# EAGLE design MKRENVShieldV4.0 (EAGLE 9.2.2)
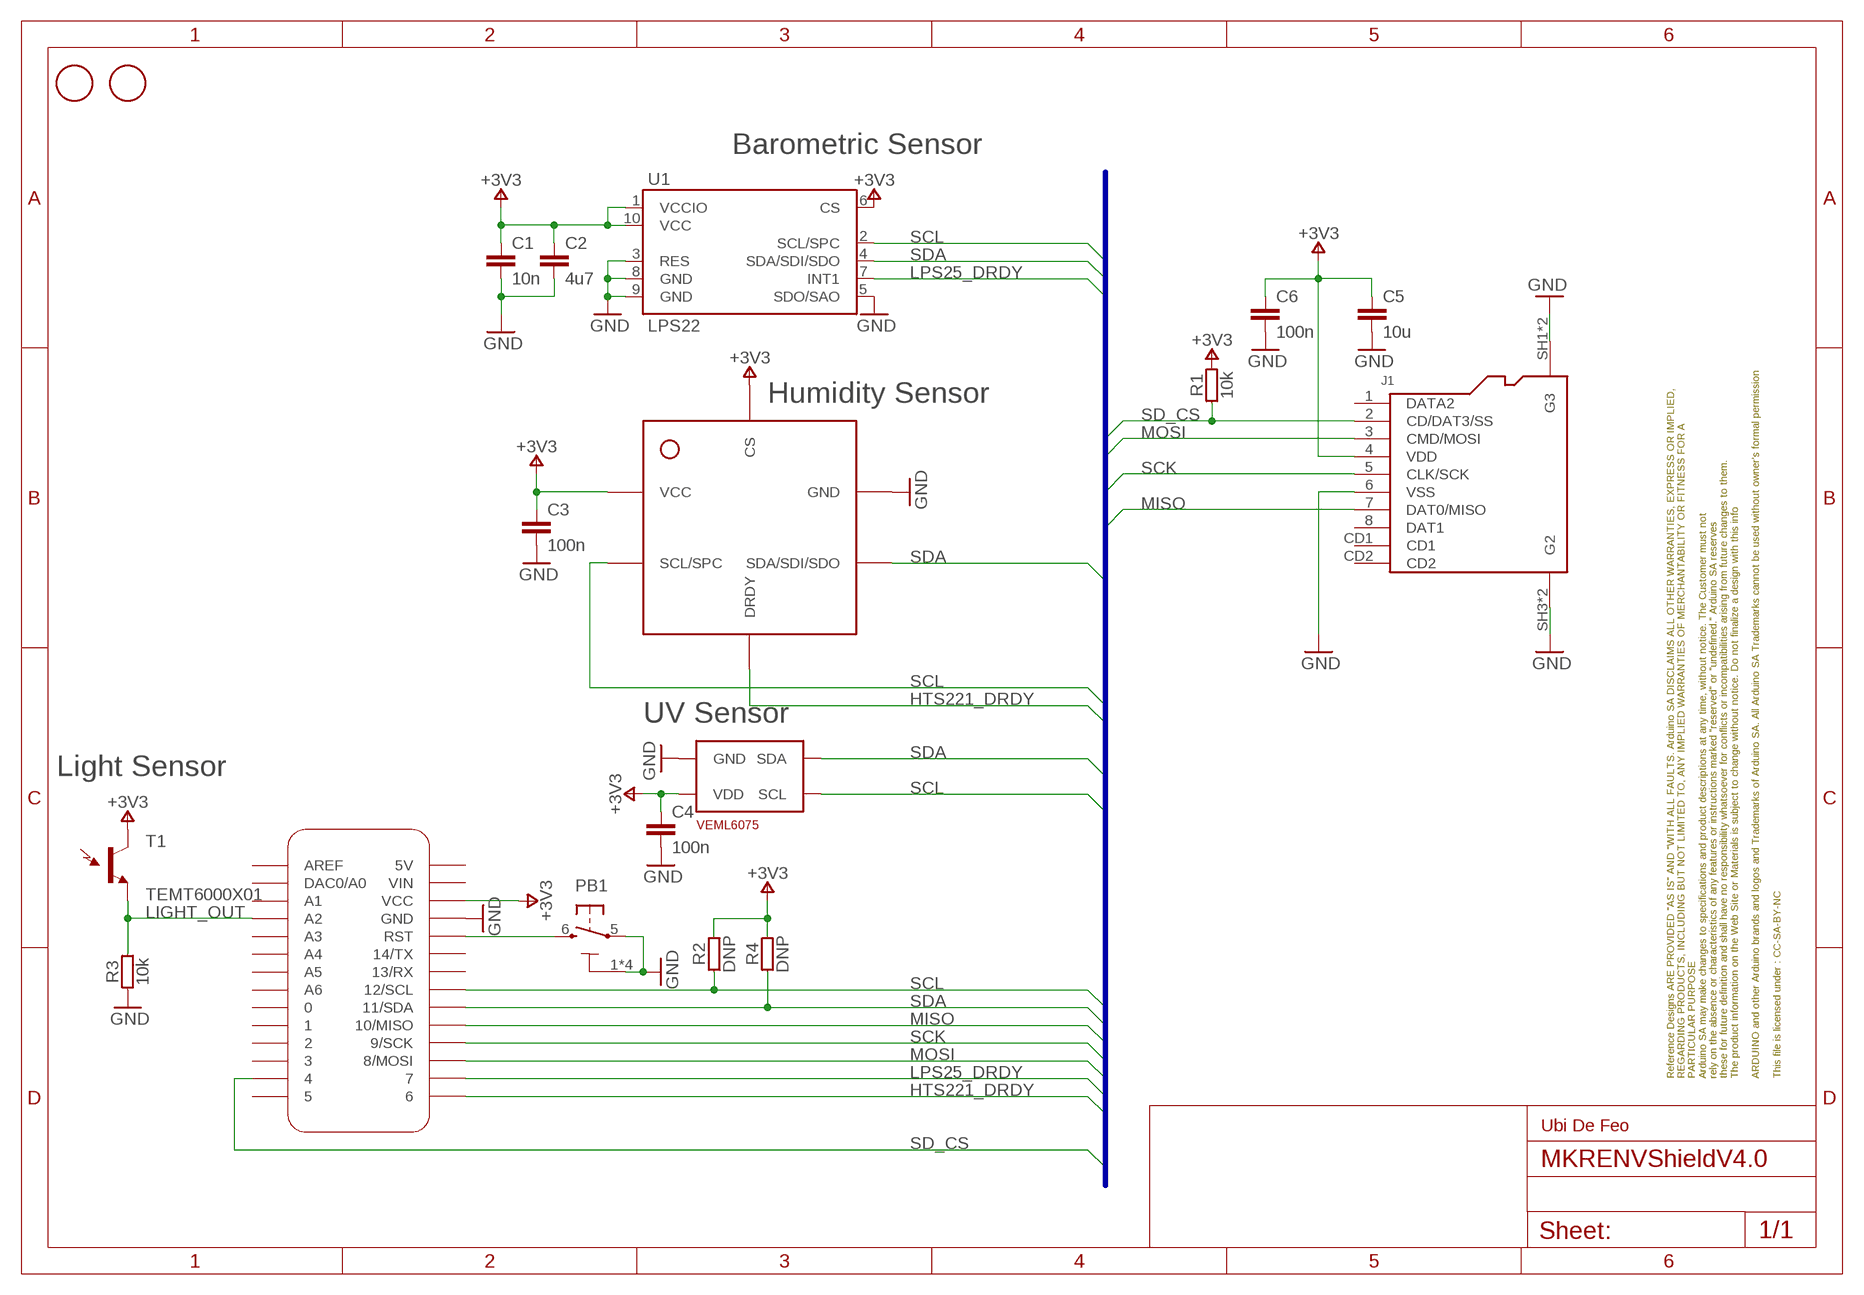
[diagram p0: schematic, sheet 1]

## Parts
C1  10n  C-10NF-0402  [0402-1005X55N]
C2  4u7  C-4.7UF-0402  [0402-1005X55N]
C3  100n  C-100NF-0402  [0402-1005X55N]
C4  100n  C-100NF-0402  [0402-1005X55N]
C5  10u  C-10UF-0603  [0603-1608X90N]
C6  100n  C-100NF-0402  [0402-1005X55N]
FD1  DNP  FIDUCIAL-1.5MM  [FD-1-1.5]
FD2  DNP  FIDUCIAL-1.5MM  [FD-1-1.5]
FRAME1  DNP  A4L-LOC  [FRAME]
J1  -  SD_AMPHENOL  [AMPHENOL_114-00841-68]
MKR1  -  MKRBOARD-SHORTTEXT  [MKRBOARD-DIM-SHORTTEXT]
PB1  PTS820  TACTILE1PTS820-NH  [C&K_PTS820_NO_HOLES]
R1  10k  R-10K-0402  [0402-1005X55N]
R2  DNP  R-DNP-0402  [0402-1005X55N]
R3  10k  R-10K-0402  [0402-1005X55N]
R4  DNP  R-DNP-0402  [0402-1005X55N]
T1  TEMT6000X01  TEMT6000  [TEMT6000-SEN]
U1  LPS22  LPS2XH-22  [LPS22H]
U2  HTS221  [HTS221]
U4  VEML6075  [VEML6075]

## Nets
+3V3: C1.1 C2.1 C3.1 C4.1 C5.1 C6.1 J1.4(VDD) MKR1.VCC R1.2 R2.2 R4.2 T1.COLLECTOR(C1) U1.1(VCCIO) U1.6(CS) U1.10(VCC) U2.P$1.VDD(VCC) U2.P$6.CS(CS) U4.P$4(VDD)
GND: C1.2 C2.2 C3.2 C4.2 C5.2 C6.2 J1.6(VSS) J1.SH1(G3) J1.SH2(G3) J1.SH3(G2) J1.SH4(G2) MKR1.GND PB1.1 PB1.2 PB1.3 PB1.4 PB1.5 R3.1 U1.3(RES) U1.5(SDO/SAO) U1.8(GND) U1.9(GND) U2.P$5.GND(GND) U4.P$1(GND)
HTS221_DRDY: MKR1.6 U2.P$3.DRDY(DRDY)
LIGHT_OUT: MKR1.A2 R3.2 T1.EMITTER(E1)
LPS25_DRDY: MKR1.7 U1.7(INT1)
MISO: J1.7(DAT0/MISO) MKR1.10(10/MISO)
MOSI: J1.3(CMD/MOSI) MKR1.8(8/MOSI)
RESET: MKR1.RST PB1.6
SCK: J1.5(CLK/SCK) MKR1.9(9/SCK)
SCL: MKR1.12(12/SCL) R2.1 U1.2(SCL/SPC) U2.P$2.SCL/SPC(SCL/SPC) U4.P$3(SCL)
SD_CS: J1.2(CD/DAT3/SS) MKR1.4 R1.1
SDA: MKR1.11(11/SDA) R4.1 U1.4(SDA/SDI/SDO) U2.P$4.SDA/SDI/SDO(SDA/SDI/SDO) U4.P$2(SDA)
Unconnected: J1.1(DATA2) J1.8(DAT1) J1.CD1 J1.CD2 MKR1.0 MKR1.1 MKR1.2 MKR1.3 MKR1.5 MKR1.5V MKR1.13(13/RX) MKR1.14(14/TX) MKR1.A0(DAC0/A0) MKR1.A1 MKR1.A3 MKR1.A4 MKR1.A5 MKR1.A6 MKR1.AREF MKR1.VIN

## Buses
HTS221_DRDY,LPS25_DRDY,MISO,MOSI,SCK,SCL,SDA,SD_CS

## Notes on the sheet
- Barometric Sensor
- Humidity Sensor
- UV Sensor
- Light Sensor
- Ubi De Feo

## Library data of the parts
C1 = Arduino-rcl:C: SMD Capacitor; CODE-ARDUINO: 0165; DATASHEET: http://search.murata.co.jp/Ceramy/image/img/A01X/partnumbering_e_01.pdf; DISTRIBUTOR-LINK: http://www.digikey.com/product-detail/en/murata-electronics-north-america/GRM155R71H103KA88J/490-6351-1-ND/3845548; DISTRIBUTOR-PN: 490-6351-1-ND; MANUFACTURER: Murata; MANUFACTURER-PN: GRM155R71H103KA88J; NOTE: -
C2 = Arduino-rcl:C: SMD Capacitor; CODE-ARDUINO: 0833; DATASHEET: http://search.murata.co.jp/Ceramy/image/img/A01X/partnumbering_e_01.pdf; DISTRIBUTOR-LINK: http://www.digikey.com/product-detail/en/murata-electronics-north-america/GRM155R60J475ME47D/490-5915-1-ND/3719860; DISTRIBUTOR-PN: 490-5915-1-ND; MANUFACTURER: Murata; MANUFACTURER-PN: GRM155R60J475ME47D; NOTE: -
C3 C4 C6 = Arduino-rcl:C: SMD Capacitor; CODE-ARDUINO: 0132; DATASHEET: http://www.tdk.com/pdf/TDKMLCCCapRange.pdf; DISTRIBUTOR-LINK: http://www.digikey.com/product-detail/en/tdk-corporation/C1005X5R1H104K050BB/445-5942-1-ND/2443982; DISTRIBUTOR-PN: 445-5942-1-ND; MANUFACTURER: TDK; MANUFACTURER-PN: C1005X5R1H104K050BB; NOTE: -
C5 = Arduino-rcl:C: SMD Capacitor; CODE-ARDUINO: 2213; DATASHEET: http://www.murata.com/~/media/webrenewal/support/library/catalog/products/capacitor/mlcc/c02e.pdf; DISTRIBUTOR-LINK: http://www.digikey.com/product-search/en?keywords=490-10728-1-ND; DISTRIBUTOR-PN: 490-10728-1-ND; MANUFACTURER: Murata; MANUFACTURER-PN: GRM188R61C106KAALD; NOTE: -
FD1 FD2 = Arduino-utility:FIDUCIAL: Fiducial mount; CODE-ARDUINO: DNP; DATASHEET: DNP; DISTRIBUTOR-LINK: DNP; DISTRIBUTOR-PN: DNP; MANUFACTURER: DNP; MANUFACTURER-PN: DNP
FRAME1 = Arduino-utility:A4L-LOC: FRAME; CODE-ARDUINO: DNP; DATASHEET: DNP; DISTRIBUTOR-LINK: DNP; DISTRIBUTOR-PN: DNP; MANUFACTURER: DNP; MANUFACTURER-PN: DNP
J1 = Arduino-connectors:SD_AMPHENOL: Micro SD connector; CODE-ARDUINO: A5328; DATASHEET: https://www.amphenolcanada.com/ProductSearch/drawings/AC/1140084168.pdf; DISTRIBUTOR-LINK: http://www.digikey.com/product-detail/en/amphenol-commercial-products/114-00841-68/114-00841-68-1-ND/2187101; DISTRIBUTOR-PN: 114-00841-68-1-ND; MANUFACTURER: Amphenol; MANUFACTURER-PN: 114-00841-68; NOTE: NO
MKR1 = Arduino-utility:MKRBOARD: MKR board footprint; CODE-ARDUINO: -; DATASHEET: -; DISTRIBUTOR-LINK: -; DISTRIBUTOR-PN: -; MANUFACTURER: -; MANUFACTURER-PN: -
PB1 = Arduino-pushbuttons:TACTILE1: Tactile Switch SPST-NO Top Actuated Surface Mount; CODE-ARDUINO: 0173; DATASHEET: http://www.ckswitches.com/media/1474/pts820.pdf; DISTRIBUTOR-LINK: https://www.digikey.com/product-detail/en/c-k/PTS820-J15M-SMTR-LFS/CKN10506CT-ND/4176681; DISTRIBUTOR-PN: PTS820 J25K SMTR LFS-ND; MANUFACTURER: C&K; MANUFACTURER-PN: PTS820 J25K SMTR LFS
R1 R3 = Arduino-rcl:R: SMD Resistor; CODE-ARDUINO: 0136; DATASHEET: www.yageo.com.tw/exep/pages/download/literatures/PYu-R_INT-thick_7.pdf; DISTRIBUTOR-LINK: http://www.digikey.com/product-detail/en/yageo/RC0402FR-0710KL/311-10.0KLRCT-ND/729470; DISTRIBUTOR-PN: 311-10.0KLRCT-ND; MANUFACTURER: Yageo; MANUFACTURER-PN: RC0402FR-0710KL; NOTE: NO
R2 R4 = Arduino-rcl:R: SMD Resistor; CODE-ARDUINO: DNP; DATASHEET: DNP; DISTRIBUTOR-LINK: DNP; DISTRIBUTOR-PN: DNP; MANUFACTURER: DNP; MANUFACTURER-PN: DNP; NOTE: NO
T1 = Arduino-Sensors:TEMT6000: Ambient Light Sensor; CODE-ARDUINO: A5355; DATASHEET: https://www.vishay.com/docs/81579/temt6000.pdf; DISTRIBUTOR-LINK: https://nl.mouser.com/ProductDetail/Vishay-Semiconductors/TEMT6000X01?qs=sGAEpiMZZMtIHXa%252bTo%2fr2WJrbra4XIks; DISTRIBUTOR-PN: 78-TEMT6000; MANUFACTURER: Vishay Semiconductors; MANUFACTURER-PN: TEMT6000X01
U1 = Arduino-Sensors:LPS2XH; CODE-ARDUINO: A5390; DATASHEET: https://www.st.com/content/ccc/resource/technical/document/datasheet/bf/c1/4f/23/61/17/44/8a/DM00140895.pdf/files/DM00140895.pdf/jcr:content/translations/en.DM00140895.pdf; DISTRIBUTOR-LINK: https://www.digikey.com/product-detail/en/stmicroelectronics/LPS22HBTR/497-16265-1-ND/5799917; DISTRIBUTOR-PN: 497-16265-1-ND; MANUFACTURER: ST; MANUFACTURER-PN: LPS22HBTR
U2 = Arduino-Sensors:HTS221; CODE-ARDUINO: A5356; DATASHEET: https://nl.mouser.com/datasheet/2/389/hts221-954783.pdf; DISTRIBUTOR-LINK: https://nl.mouser.com/ProductDetail/STMicroelectronics/HTS221TR?qs=%2fha2pyFaduhYqhgVSCoMJjbIcKdCD1D5p03chi4OA3k%3d; DISTRIBUTOR-PN: 511-HTS221TR; MANUFACTURER: STMicroelectronics; MANUFACTURER-PN: HTS221TR
U4 = Arduino-Sensors:VEML6075: The VEML6075 senses UVA and UVB light and incorporates photodiode, amplifiers, and analog / digital circuits into a single chip using a CMOS process. When the UV sensor is applied, it is able to detect UVA and UVB intensity to provide a measure of the signal strength as well as allowing for UVI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; CODE-ARDUINO: A5354; DATASHEET: http://www.vishay.com/docs/84304/veml6075.pdf; DISTRIBUTOR-LINK: https://www.digikey.com/product-detail/en/vishay-semiconductor-opto-division/VEML6075/VEML6075CT-ND/5878946; DISTRIBUTOR-PN: VEML6075CT-ND; MANUFACTURER: Vishay Semiconductor Opto Division; MANUFACTURER-PN: VEML6075

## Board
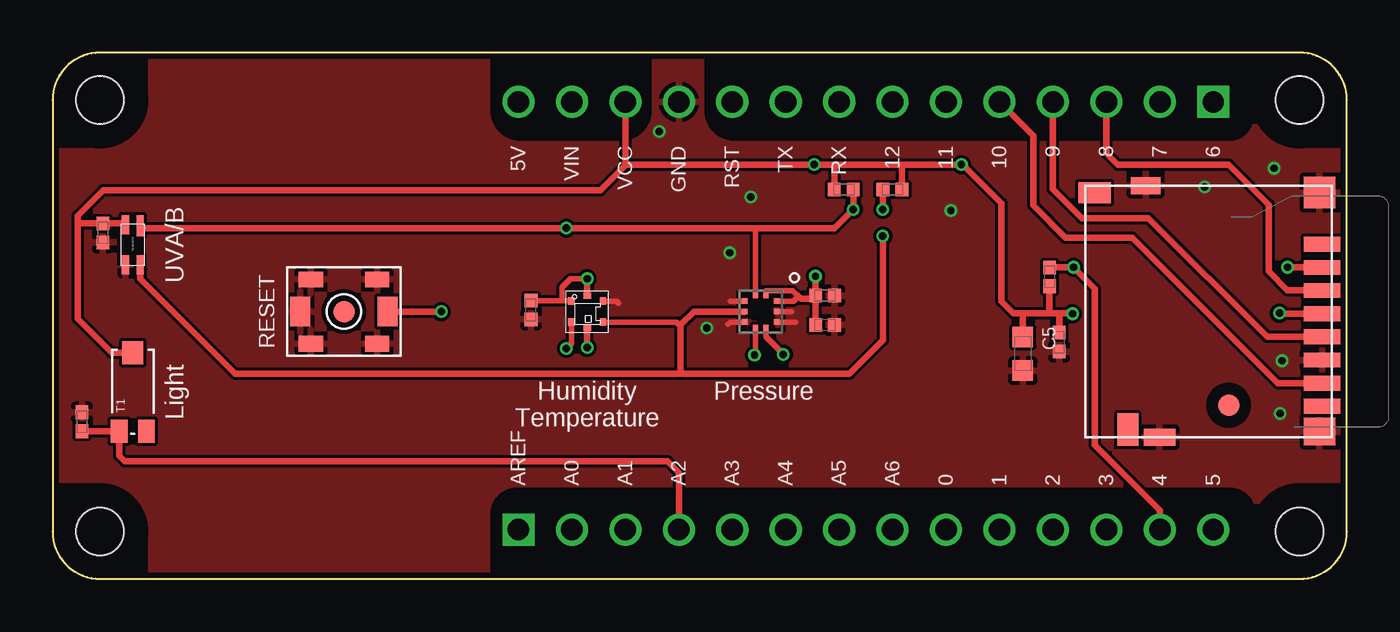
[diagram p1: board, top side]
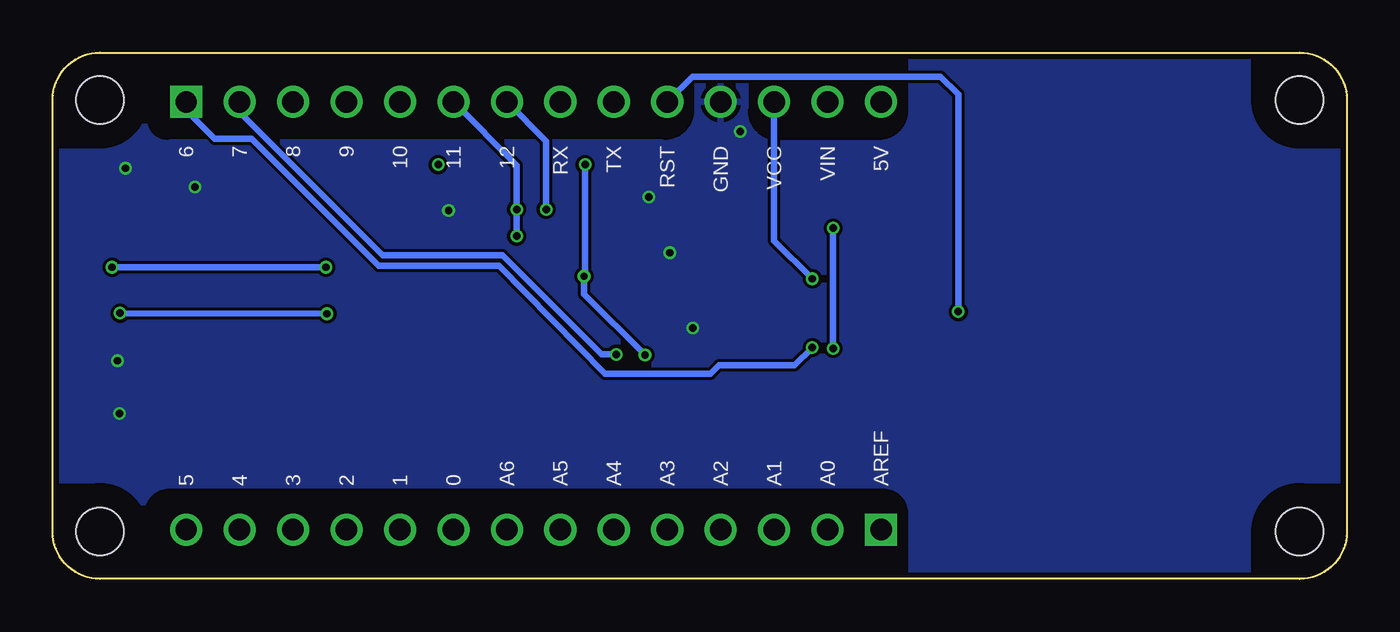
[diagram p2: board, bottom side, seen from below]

Size 61.5 x 25 mm. Coordinates in mm from the lower left corner, seen from the top.
Copper layers (1*16): Top 0.018mm / dielectric 1.55mm / Bottom 0.018mm
Design rules "eC_2Layer_PClass6_BaseCopperO18_eCDefault": minimum track width 0.15mm, minimum drill 0.35mm, track to track 0.15mm, track to pad 0.15mm, pad to pad 0.15mm, via to via 0.15mm, smd to smd 0mil, copper to edge 0.25mm, drill to drill 0.35mm, minimum pad ring 0.175mm, minimum via ring 0.125mm, stop-mask expansion 0mil, vias tented up to drill 0.45mm, thermal gap 0.2mm
tRestrict: area 33.2,12.3 to 34.1,13.1; area 32.5,13 to 33.1,13.7; area 32.5,11.7 to 33,12.3; area 24.4,11.7 to 26.4,13.7; area 3.1,14.9 to 4.4,16.9; 19 lines
bRestrict: 16 lines

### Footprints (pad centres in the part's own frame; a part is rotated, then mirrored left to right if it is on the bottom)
0402-1005X55N = smd 0.62 x 0.62: 1 -0.45,0; 2 0.45,0
0603-1608X90N = smd 0.95 x 1: 1 -0.8,0; 2 0.8,0
FD-1-1.5 = smd 1.016 x 1.016: P$1 0,0
AMPHENOL_114-00841-68 = smd 0.7 x 1.75: 1 3.2,-5.888; 2 2.1,-5.888; 3 1,-5.888; 4 -0.1,-5.888; 5 -1.2,-5.888; 6 -2.3,-5.888; 7 -3.4,-5.888; 8 -4.5,-5.888 | smd 1 x 1.55: CD1 5.65,4.912 | smd 1.55 x 1: CD2 -5.602,3.337 | smd 1.3 x 1.5: SH1 -5.7,-5.76 | smd 1.5 x 1.5: SH2 5.65,-5.76 | smd 0.8 x 1.4: SH3 5.975,2.487 | smd 0.8 x 1.5: SH4 -5.975,1.837
MKRBOARD-DIM-SHORTTEXT = drill 1.016 pad 1.524: 0 42.455,2.34; 1 44.995,2.34; 2 47.535,2.34; 3 50.075,2.34; 4 52.615,2.34; 5 55.155,2.34; 5V 22.135,22.66; 7 52.615,22.66; 8 50.075,22.66; 9 47.535,22.66; 10 44.995,22.66; 11 42.455,22.66; 12 39.915,22.66; 13 37.375,22.66; 14 34.835,22.66; A0 24.675,2.34; A1 27.215,2.34; A2 29.755,2.34; A3 32.295,2.34; A4 34.835,2.34; A5 37.375,2.34; A6 39.915,2.34; GND 29.755,22.66; RST 32.295,22.66; VCC 27.215,22.66; VIN 24.675,22.66 | drill 1.016 pad 1.524 square: 6 55.155,22.66; AREF 22.135,2.34 | hole 2.25: 59.25,2.25; 59.25,22.75; 2.25,2.25; 2.25,22.75
C&K_PTS820_NO_HOLES = smd 1.15 x 0.75: 1 -1.575,1.525; 2 -1.575,-1.525; 3 1.575,1.525; 4 1.575,-1.525 | smd 0.95 x 1.4: 5 -2.075,0; 6 2.075,0
TEMT6000-SEN = smd 1.1 x 0.8: BASE -1.87,-0.65; EMITTER -1.87,0.65 | smd 1.1 x 1: COLLECTOR 1.86,0.01
LPS22H = smd 0.25 x 0.275: 1 -0.25,-0.762; 2 0.25,-0.762; 6 0.25,0.762; 7 -0.25,0.762 | smd 0.275 x 0.25: 3 0.762,-0.5; 4 0.762,0; 5 0.762,0.5; 8 -0.762,0.5; 9 -0.762,0; 10 -0.762,-0.5
HTS221 = smd 0.3 x 0.35: P$1.VDD -0.75,0.5; P$2.SCL/SPC -0.75,-0.5; P$4.SDA/SDI/SDO 0.75,-0.5; P$5.GND 0.75,0.5 | smd 0.35 x 0.3: P$3.DRDY 0,-0.75; P$6.CS 0,0.75
VEML6075 = smd 0.9 x 0.35: P$1 -0.95,0.35; P$2 -0.95,-0.35; P$4 0.95,0.35 | smd 1 x 0.35: P$3 0.9,-0.35

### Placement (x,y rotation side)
C1  36.7,12.06 0 top
C2  36.7,13.46 0 top
C3  22.73,12.78 270 top
C4  2.39,16.43 270 top
C5  46.1,10.69 270 top
C6  47.83,11.25 270 top
FD1  13.84,12.7 0 top
FD2  55.88,8.26 0 top
FRAME1  not placed on the board
J1  54.43,12.7 90 top
MKR1  0,0 0 top
PB1  13.84,12.7 0 top
R1  47.37,14.35 270 top
R2  37.59,18.49 180 top
R3  1.4,7.47 270 top
R4  39.9,18.49 0 top
T1  3.81,8.89 90 top
U1  33.65,12.7 180 top
U2  25.4,12.7 0 top
U4  3.81,15.88 90 top

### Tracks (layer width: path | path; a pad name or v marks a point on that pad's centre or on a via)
+3V3  (via drill 0.35, 0.35 pad 0.25)
  Top 0.254: U1.6 33.4,10.68 v33.35,10.64 | U1.10 35.21,13.2 35.43,13.43 35.16,13.7 33.9,13.7 U1.1 | 24.2,13.23 C3.1 22.73,13.39 | 24.2,13.23 24.62,13.23 U2.P$1.VDD | v25.4,14.26 24.6,14.26 24.2,13.86 24.2,13.23
  Top 0.305: C2.1 36.09,13.3 35.56,13.3 35.43,13.43 | C1.1 C2.1 | C2.1 v36.25,14.38 | 37.08,19.68 v36.2,19.68 27.25,19.68 | 37.08,19.68 40.39,19.68 | 40.39,19.68 v43.18,19.68 43.25,19.68 45.09,17.85 45.09,13.18 45.64,12.62 46.1,12.62 | 47.83,12.62 47.45,12.62 | MKR1.VCC 27.21,19.72 27.25,19.68 | T1.COLLECTOR 2.81,10.75 1.19,12.37 1.19,16.87 | U2.P$6.CS v25.4,14.26 | J1.4 58.32,12.6 v58.29,12.62 | R2.2 37.14,19.63 37.08,19.68 | R4.2 40.35,19.65 40.39,19.68 | 27.25,19.68 26.04,18.47 2.42,18.47 1.19,17.25 1.19,16.87 | 1.19,16.87 1.21,16.88 C4.1 3.4,16.88 U4.P$4 | C6.1 47.83,12.62 | R1.2 47.37,12.7 47.45,12.62 | 47.45,12.62 46.1,12.62 | C5.1 46.1,12.62 | 47.83,12.62 48.44,12.62 v48.46,12.6
  Bottom 0.305: v48.46,12.6 v58.29,12.62 | v33.35,10.64 36.25,13.53 v36.25,14.38 36.2,14.43 v36.2,19.68 | v25.4,14.26 27.21,16.07 MKR1.VCC
GND  (via drill 0.35)
  Top 0.254: U1.8 35.3,12.2 | U1.9 35.1,12.7 | U1.3 32.2,13.2 | U1.5 32.2,12.2 32.1,12.1 | U2.P$5.GND 26.8,13.2 26.9,13.1
  other vias: 31.09,11.91 28.83,21.26 54.74,18.62 32.18,15.49 58.04,19.51 58.42,10.36 33.17,18.14 42.68,17.49 58.32,7.86
  pour Top: 2.54,25.02 59.18,25.02 arc-90 61.72,22.48 61.72,2.54 arc-90 59.18,0 2.54,0 arc-90 0,2.54 0,22.48 arc-90
  pour Bottom: 2.54,25.02 59.18,25.02 arc-90 61.72,22.48 61.72,2.54 arc-90 59.18,0 2.54,0 arc-90 0,2.54 0,22.48 arc-90
HTS221_DRDY  (via drill 0.35)
  Top 0.305: U2.P$3.DRDY v25.4,10.99
  Bottom 0.305: MKR1.6 55.16,22.27 53.81,20.92 52.03,20.92 46,14.89 40.29,14.89 35.26,9.73 30.23,9.73 29.83,10.14 26.25,10.14 v25.4,10.99
LIGHT_OUT
  Top 0.305: R3.2 T1.EMITTER 3.16,5.86 3.43,5.59 29.21,5.59 29.75,5.04 MKR1.A2
LPS25_DRDY  (via drill 0.35)
  Top 0.254: U1.7 33.9,11.49 v34.72,10.67
  Bottom 0.305: v34.72,10.67 35.42,10.67 40.13,15.38 45.83,15.38 52.62,22.16 MKR1.7
MISO
  Top 0.305: MKR1.10 46.6,21.06 46.6,17.75 48.13,16.21 51.31,16.21 58.22,9.3 J1.7
MOSI
  Top 0.305: MKR1.8 50.08,20.23 50.62,19.68 55.88,19.68 57.78,17.78 57.78,14.61 58.67,13.72 60.3,13.72 J1.3
RESET  (via drill 0.35)
  Top 0.305: PB1.6 v18.47,12.7
  Bottom 0.305: v18.47,12.7 18.47,23.01 19.3,23.85 31.1,23.85 MKR1.RST
SCK
  Top 0.305: MKR1.9 47.53,18.5 48.9,17.14 52.07,17.14 57.72,11.5 J1.5
SCL  (via drill 0.35)
  Top 0.254: U1.2 33.4,16.62 33.35,16.66 | U2.P$2.SCL/SPC 24.65,11.19 v24.41,10.95
  Top 0.305: R2.1 v38.04,17.56 | v38.04,17.56 v38.05,17.55 | 33.35,16.66 v24.41,16.66 4.27,16.66 U4.P$3 | 33.35,16.66 37.15,16.66 v38.04,17.56 | 33.35,16.66
  Bottom 0.305: MKR1.12 38.05,20.79 v38.05,17.55 | v24.41,16.66 v24.41,10.95
SD_CS  (via drill 0.35)
  Top 0.305: R1.1 v48.51,14.81 49.53,13.79 49.53,6.35 52.62,3.27 MKR1.4 | J1.2 58.68,14.8 v58.67,14.81
  Bottom 0.305: v58.67,14.81 v48.51,14.81
SDA  (via drill 0.35)
  Top 0.254: 29.84,12 29.64,12.2 U2.P$4.SDA/SDI/SDO
  Top 0.305: U1.4 30.48,12.7 29.84,12.06 29.84,12 29.84,9.79 29.8,9.74 | v39.45,16.28 39.47,16.26 39.47,11.34 37.87,9.73 29.83,9.73 29.83,9.74 29.8,9.74 | R4.1 v39.45,17.55 | U4.P$2 4.16,14.26 8.67,9.74 29.8,9.74
  Bottom 0.305: MKR1.11 39.45,19.65 v39.45,17.55 v39.45,16.28

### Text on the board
tPlace: UVA/B | RESET | Light | Humidity | Pressure | Temperature

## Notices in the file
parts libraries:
Arduino-utility: Copyright (c) 2016-2017 Arduino LLC. All right reserved.
Arduino-utility: This file is licensed under : CC-SA-BY-NC
